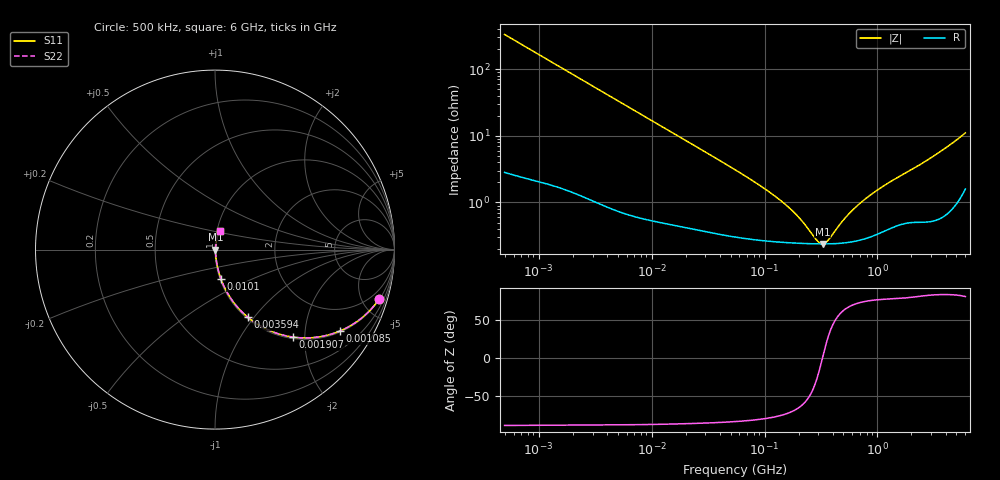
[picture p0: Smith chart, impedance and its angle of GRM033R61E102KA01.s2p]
!Murata Part Number: GRM033R61E102KA01
!These Parameters are Measured in Series Mode Connection
!  o--ll--o
!Port1  Port2
!  o------o
!Operation Temp=25[C], DC Bias Voltage=0[V]
!Freq. Start=500[kHz] Stop=6000000[kHz] 401[Steps]
# Hz S RI R 50
!Freq.(Hz) S11(Real) S11(Imag) S21(Real) S21(Imag) S12(Real) S12(Imag) S22(Real) S22(Imag)
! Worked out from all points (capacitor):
!   401 points, 500 kHz to 6 GHz, reference 50 ohm
!   read as one part in series: C = 963 pF near 524 kHz
!   lowest |Z| = 239 mohm at 326.3 MHz (marker M1)
!   series resonance near 325.7 MHz, so ESL is about 250 pH
!   S11 on the Smith chart (normalised r, x): 500 kHz: 1.06, -6.61; 1.085 MHz: 1.04, -3.06; 1.907 MHz: 1.03, -1.75; 3.594 MHz: 1.02, -0.93; 10.1 MHz: 1.01, -0.33; 6 GHz: 1.03, +0.22
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500000  0.9141 -0.276  0.0859 0.276  0.0859 0.276  0.9141 -0.276
745307  0.8287 -0.3715  0.1713 0.3715  0.1713 0.3715  0.8287 -0.3715
1085182  0.6978 -0.4528  0.3022 0.4528  0.3022 0.4528  0.6978 -0.4528
1906573  0.4344 -0.4874  0.5656 0.4874  0.5656 0.4874  0.4344 -0.4874
2411198  0.3275 -0.4604  0.6725 0.4604  0.6725 0.4604  0.3275 -0.4604
3594165  0.1838 -0.3776  0.8162 0.3776  0.8162 0.3776  0.1838 -0.3776
5748534  0.0843 -0.2665  0.9157 0.2665  0.9157 0.2665  0.0843 -0.2665
1.009969e7  0.0321 -0.1612  0.9679 0.1612  0.9679 0.1612  0.0321 -0.1612
1.162775e7  0.0255 -0.1412  0.9745 0.1412  0.9745 0.1412  0.0255 -0.1412
2.297399e7  0.00939 -0.0732  0.9906 0.0732  0.9906 0.0732  0.00939 -0.0732
5.477226e7  0.00396 -0.0306  0.996 0.0306  0.996 0.0306  0.00396 -0.0306
1.468502e8  0.0026 -0.00953  0.9974 0.00953  0.9974 0.00953  0.0026 -0.00953
1.992728e8  0.00247 -0.00554  0.9975 0.00554  0.9975 0.00554  0.00247 -0.00554
2.641335e8  0.0024 -0.0023  0.9976 0.0023  0.9976 0.0023  0.0024 -0.0023
2.970388e8  0.00239 -0.00101  0.9976 0.00101  0.9976 0.00101  0.00239 -0.00101
3.26291e8  0.00238 2.14e-05  0.9976 -2.14e-05  0.9976 -2.14e-05  0.00238 2.14e-05
3.669398e8  0.00239 0.00131  0.9976 -0.00131  0.9976 -0.00131  0.00239 0.00131
4.979299e8  0.00248 0.00482  0.9975 -0.00482  0.9975 -0.00482  0.00248 0.00482
6.446822e8  0.00269 0.00812  0.9973 -0.00812  0.9973 -0.00812  0.00269 0.00812
1.273756e9  0.00437 0.0195  0.9956 -0.0195  0.9956 -0.0195  0.00437 0.0195
2.830198e9  0.00699 0.0435  0.993 -0.0435  0.993 -0.0435  0.00699 0.0435
6e9  0.027 0.1048  0.973 -0.1048  0.973 -0.1048  0.027 0.1048
